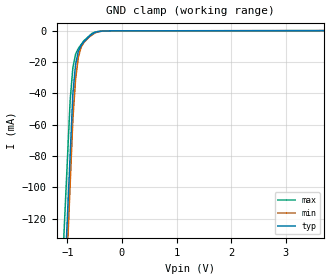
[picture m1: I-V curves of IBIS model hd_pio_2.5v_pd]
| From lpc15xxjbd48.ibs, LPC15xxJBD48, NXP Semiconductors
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[Model] hd_pio_2.5v_pd
Model_type Input
Vinl = 990.000mV
Vinh = 2.31000V
C_comp 598.000fF 598.000fF 598.000fF
| variable typ   min   max
[Voltage Range] 2.50000V 2.25000V 2.75000V
[POWER Clamp Reference] 2.50000V 2.25000V 2.75000V
[GND Clamp Reference] 0.00000V 0.00000V 0.00000V
[Temperature Range]   25   85   -40
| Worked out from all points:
|   GND clamp passes 1 mA (typ) near -0.48 V on its own axis
[GND Clamp]
-2.5V     -1.297A    -1.397A    -1.21A
-950mV    -79.19mA   -98.06mA   -44.3mA
-900mV    -39.9mA    -56.15mA   -23.45mA
-850mV    -21.32mA   -30.65mA   -14.91mA
-800mV    -13.08mA   -16.85mA   -11.27mA
-750mV    -9.388mA   -10.56mA   -8.854mA
-700mV    -7.009mA   -7.52mA    -6.441mA
-550mV    -2.202mA   -2.697mA   -1.729mA
-500mV    -1.235mA   -1.476mA   -937.3uA
-400mV    -339.6uA   -408.3uA   -368.1uA
-175mV    -30.66uA   -49.22uA   -31.16uA
5V        116.8uA    125.7uA    112.4uA
[POWER Clamp]
-2.5V     0A         0A         0A
5V        0A         0A         0A
